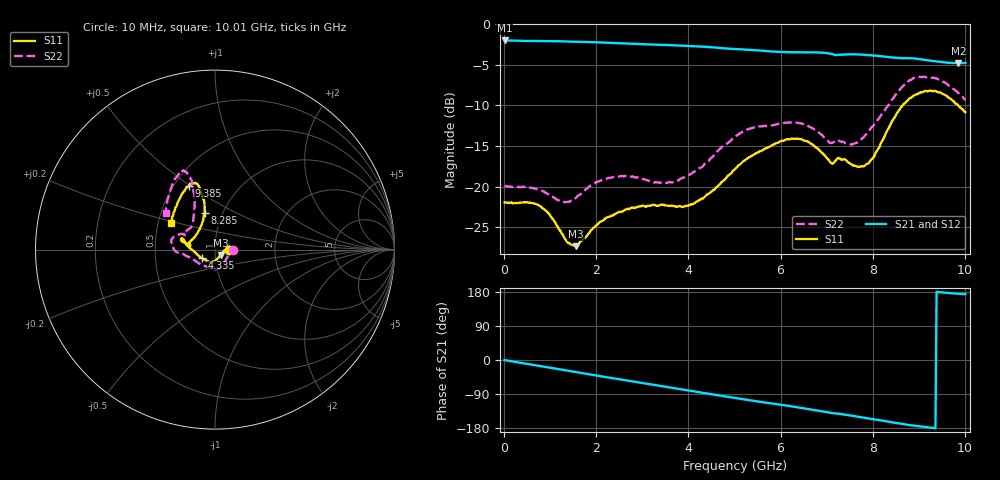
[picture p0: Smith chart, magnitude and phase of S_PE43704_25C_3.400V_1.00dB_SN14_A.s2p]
! Device ID: PE43704
! Dir: z:\PE43704\PE43704_Char_1_20130516\PE43704\AMB\3p400V\1p00dB
! Serial: 14
! Insertion: A
! Impedance: 50 ohm
! Temp: Amb
! VDD: 3.400V
! Attenuation Step: 1.00dB
! IDD: 1.140682e-01mA
#  Hz  S  RI  R  50
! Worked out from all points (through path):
!   401 points, 10 MHz to 10.01 GHz, reference 50 ohm
!   highest |S21| = -2.00 dB at 10 MHz (marker M1); lowest = -4.8 dB at 9.86 GHz (marker M2)
!   group delay of S21, straight-line fit = 53 ps
!   lowest |S11| = -27.3 dB at 1.56 GHz (marker M3), VSWR 1.09, Z = 53.1 - j3.21 ohm
!   |S11| at or under -10 dB: start of sweep to 8.647 GHz; 9.851 GHz to end of sweep
!   |S22| runs from -21.9 to -6.5 dB; largest |S21 - S12| = 0.0059
!   S11 on the Smith chart (normalised r, x): 10 MHz: 1.17, +0.00; 4.335 GHz: 0.86, -0.08; 8.285 GHz: 0.82, +0.35; 9.385 GHz: 0.59, +0.50; 10.01 GHz: 0.58, +0.19
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1e7  0.0801 0.000294  0.7939 -0.0032  0.7941 -0.00301  0.1011 0.000103
7.6e8  0.0737 0.0216  0.7582 -0.2112  0.7582 -0.2112  0.0953 0.00751
1.285e9  0.0494 -0.00785  0.7027 -0.3474  0.7026 -0.3473  0.073 -0.0343
1.56e9  0.0308 -0.0302  0.6628 -0.413  0.6626 -0.4132  0.0569 -0.064
1.685e9  0.0231 -0.0407  0.6421 -0.4417  0.642 -0.4417  0.0482 -0.0777
2.41e9  -0.0122 -0.0669  0.5006 -0.5788  0.501 -0.5781  0.0046 -0.1151
3.36e9  -0.0247 -0.0728  0.2824 -0.6915  0.283 -0.6911  -0.0326 -0.1011
3.91e9  -0.0438 -0.0616  0.1447 -0.7219  0.1453 -0.722  -0.081 -0.0808
4.335e9  -0.0706 -0.0487  0.0363 -0.7257  0.0365 -0.7259  -0.1265 -0.0511
5.01e9  -0.1285 -0.00123  -0.1235 -0.6923  -0.1232 -0.6925  -0.2019 -0.0191
6.06e9  -0.1814 0.0606  -0.3268 -0.5897  -0.3251 -0.5897  -0.2433 0.0425
6.685e9  -0.1779 0.0419  -0.4401 -0.5061  -0.4405 -0.5054  -0.2158 0.0787
7.085e9  -0.1384 0.027  -0.4982 -0.4305  -0.5004 -0.4314  -0.1676 0.0805
7.285e9  -0.1464 0.0304  -0.5115 -0.3981  -0.5101 -0.3991  -0.1622 0.1002
7.76e9  -0.1045 0.0838  -0.5699 -0.3103  -0.5692 -0.3119  -0.1232 0.1541
7.985e9  -0.0822 0.1243  -0.5866 -0.2634  -0.5866 -0.2665  -0.1177 0.2019
8.285e9  -0.0581 0.2053  -0.5968 -0.2001  -0.5955 -0.2036  -0.1141 0.2809
8.36e9  -0.0571 0.2266  -0.5993 -0.1828  -0.598 -0.1858  -0.1152 0.3036
8.835e9  -0.0859 0.3426  -0.611 -0.0821  -0.6067 -0.0831  -0.1567 0.4268
9.385e9  -0.1457 0.3565  -0.5899 0.00258  -0.591 0.00453  -0.2079 0.4121
9.86e9  -0.2238 0.2194  -0.5738 0.0519  -0.5724 0.0528  -0.266 0.2658
1.001e10  -0.2451 0.1505  -0.575 0.0628  -0.5785 0.0624  -0.2742 0.2046
